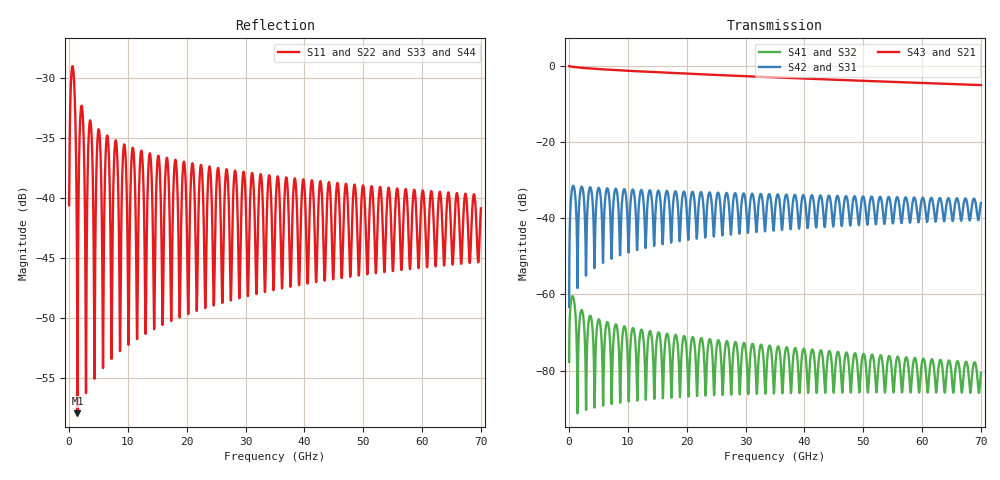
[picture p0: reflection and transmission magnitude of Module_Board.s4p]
! AWR Design Environment (8415) Thu Oct 18 13:44:33 2018
! Document = 'Module PCB'
! nPorts: 4, nXvals: 7001
# HZ S DB R 50
!Freq DBS11 AngS11 DBS12 AngS12 DBS13 AngS13 DBS14 AngS14
!	DBS21 AngS21 DBS22 AngS22 DBS23 AngS23 DBS24 AngS24
!	DBS31 AngS31 DBS32 AngS32 DBS33 AngS33 DBS34 AngS34
!	DBS41 AngS41 DBS42 AngS42 DBS43 AngS43 DBS44 AngS44
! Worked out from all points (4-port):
!   7000 points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, 10 MHz to 70 GHz, reference 50 ohm
!   strongest paths, dB at 10 MHz, 17.51 GHz, 35.01 GHz, 52.51 GHz, 70 GHz:
!     S43: -0.1, -1.9, -3.0, -4.1, -5.0
!     S21: -0.1, -1.9, -3.0, -4.1, -5.0
!     S42: -63.3, -41.2, -38.1, -36.6, -36.0
!     S31: -63.3, -41.2, -38.1, -36.6, -36.0
!     S41: -77.7, -81.7, -80.4, -80.2, -80.7
!     S32: -77.7, -81.7, -80.4, -80.2, -80.7
!   lowest |S11| = -58.0 dB at 1.43 GHz (marker M1), VSWR 1.00, Z = 50.1 - j0.0636 ohm
!   |S11| at or under -10 dB: start of sweep to end of sweep
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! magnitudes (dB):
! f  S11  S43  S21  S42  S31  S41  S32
! 10 MHz  -40.6  -0.1  -0.1  -63.3  -63.3  -77.7  -77.7
! 580 MHz  -29.0  -0.2  -0.2  -31.8  -31.8  -60.5  -60.5
! 1.43 GHz  -58.0  -0.4  -0.4  -58.3  -58.3  -89.7  -89.7
! 2.15 GHz  -32.3  -0.5  -0.5  -31.7  -31.7  -64.1  -64.1
! 2.85 GHz  -53.9  -0.6  -0.6  -52.7  -52.7  -84.6  -84.6
! 7.22 GHz  -53.4  -1.0  -1.0  -50.6  -50.6  -87.6  -87.6
! 70 GHz  -40.9  -5.0  -5.0  -36.0  -36.0  -80.7  -80.7
